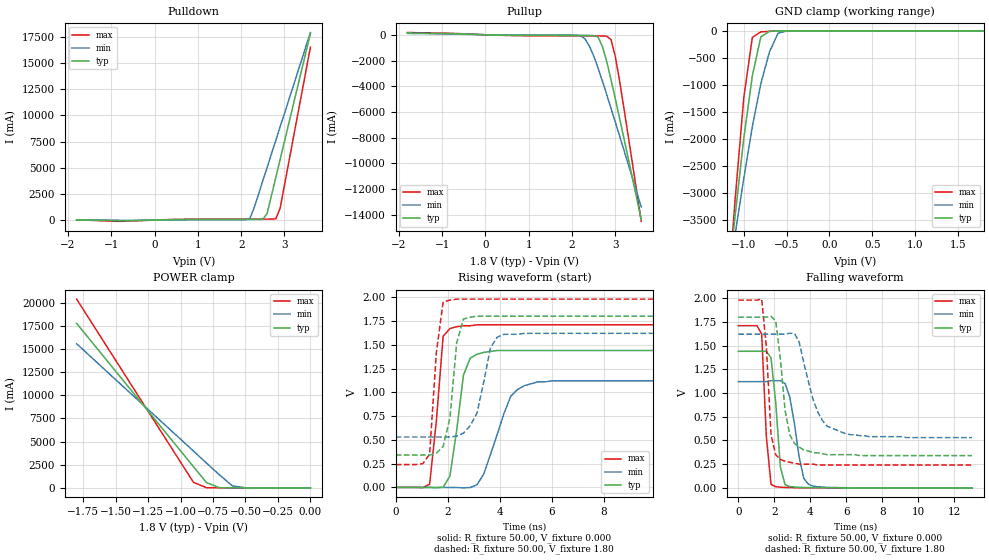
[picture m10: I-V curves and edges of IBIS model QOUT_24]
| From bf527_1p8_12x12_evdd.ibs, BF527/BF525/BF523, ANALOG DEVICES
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|   Model prw1624cdg_25
[Model]   QOUT_24
Model_type   I/O
Polarity   Non-Inverting
Enable   Active-Low
Vinl =   0.70V
Vinh =   1.00V
Vmeas =   1.20V
Cref =  50.00pF
Rref =   1.00M
Vref =  0.000V
C_comp   4.39pF   3.96pF   4.83pF
[Temperature Range]   25.00   0.12k   -40.00
[Voltage Range]   1.80V   1.62V   1.98V
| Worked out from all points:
|   slope of the pulldown table from 0 to 0.27 V, typ, clamps not added: 11.3 ohm
|   slope of the pullup table from 0 to 0.27 V, typ, clamps not added: 11.8 ohm
|   GND clamp passes 1 mA (typ) near -0.53 V on its own axis
|   POWER clamp passes 1 mA (typ) near -0.53 V on its own axis
|   rising waveform, R_fixture 50.00, V_fixture 0.000: 20-80 % time 416ps typ, 844ps min, 335ps max; typ from 0 V to 1.44 V
|   rising waveform, R_fixture 50.00, V_fixture 1.80: 20-80 % time 341ps typ, 535ps min, 306ps max; typ from 0.34 V to 1.8 V
|   falling waveform, R_fixture 50.00, V_fixture 0.000: 20-80 % time 373ps typ, 580ps min, 302ps max; typ from 1.44 V to 0 V
|   falling waveform, R_fixture 50.00, V_fixture 1.80: 20-80 % time 544ps typ, 1.03ns min, 326ps max; typ from 1.8 V to 0.34 V
[Pulldown]
| voltage   I(typ)   I(min)   I(max)
-1.8V     -10mA      0A         -10mA
-800mV    -73.8mA    -22.2mA    -120mA
600mV     42.5mA     23.13mA    69.61mA
2.1V      51.24mA    33.46mA    88.37mA
2.2V      51.32mA    140mA      88.44mA
2.3V      51.78mA    1.16A      88.5mA
2.5V      68.44mA    3.74A      89.43mA
2.6V      620mA      5.02A      92.15mA
2.8V      4.05A      7.6A       110mA
2.9V      5.77A      8.89A      1.11A
3.6V      17.82A     17.91A     16.51A
[Pullup]
| voltage   I(typ)   I(min)   I(max)
-1.8V     140mA      110mA      170mA
2.2V      -52.05mA   -57.07mA   -84.56mA
2.3V      -52.58mA   -320mA     -84.78mA
2.4V      -54.8mA    -870mA     -85.04mA
2.5V      -62.21mA   -1.62A     -86.03mA
2.6V      -160mA     -2.56A     -89.83mA
2.7V      -880mA     -3.57A     -96.83mA
2.8V      -2.04A     -4.62A     -110mA
2.9V      -3.46A     -5.69A     -360mA
3V        -4.95A     -6.77A     -1.66A
3.1V      -6.49A     -7.86A     -3.59A
3.6V      -14.34A    -13.37A    -14.49A
[GND_clamp]
| voltage   I(typ)   I(min)   I(max)
-1.8V     -14.28A    -11.35A    -18.41A
-1.2V     -4.9A      -4.81A     -5.19A
-1.1V     -3.4A      -3.75A     -3.1A
-1V       -1.99A     -2.73A     -1.24A
-900mV    -830mA     -1.77A     -120mA
-800mV    -110mA     -970mA     -19.15mA
-700mV    -9.85mA    -390mA     -9.73mA
-600mV    -2.55mA    -42.82mA   -3.48mA
-500mV    -450uA     -4.35mA    -550uA
1.8V      150pA      1.58uA     73.18pA
[POWER_clamp]
| voltage   I(typ)   I(min)   I(max)
-1.8V     17.76A     15.56A     20.38A
-900mV    2.28A      3.97A      590mA
-800mV    570mA      2.68A      16.99mA
-700mV    17.03mA    1.4A       7.08mA
-600mV    2.36mA     210mA      2.77mA
-500mV    460uA      11.86mA    530uA
0V        150pA      7.78nA     85.42pA
[Ramp]
| variable   typ   min   max
dV/dt_r   0.86/0.39n   0.67/0.76n   1.02/0.25n
dV/dt_f   0.87/0.47n   0.65/0.92n   1.04/0.28n
R_load = 50.00
[Rising Waveform]
R_fixture = 50.00
V_fixture = 0.000
V_fixture_min = 0.000
V_fixture_max = 0.000
L_fixture = 0.000H
C_fixture = 0.000F
| time   V(typ)   V(min)   V(max)
0s        0V         0V         0V
1.3ns     -450uV     54.95uV    33.4mV
1.56ns    -3.61mV    44.05uV    700mV
1.82ns    1.42mV     -63.47uV   1.59V
2.08ns    120mV      -450uV     1.67V
2.6ns     1.18V      -4.67mV    1.7V
3.12ns    1.4V       27.95mV    1.71V
4.42ns    1.44V      960mV      1.71V
4.94ns    1.44V      1.07V      1.71V
13ns      1.44V      1.12V      1.71V
[Rising Waveform]
R_fixture = 50.00
V_fixture = 1.80
V_fixture_min = 1.62
V_fixture_max = 1.98
L_fixture = 0.000H
C_fixture = 0.000F
| time   V(typ)   V(min)   V(max)
0s        340mV      530mV      240mV
1.3ns     340mV      530mV      350mV
1.56ns    360mV      530mV      1.42V
1.82ns    430mV      530mV      1.95V
2.34ns    1.52V      540mV      1.98V
2.6ns     1.77V      570mV      1.98V
3.12ns    1.8V       780mV      1.98V
3.64ns    1.8V       1.47V      1.98V
4.16ns    1.8V       1.61V      1.98V
13ns      1.8V       1.62V      1.98V
[Falling Waveform]
R_fixture = 50.00
V_fixture = 0.000
V_fixture_min = 0.000
V_fixture_max = 0.000
L_fixture = 0.000H
C_fixture = 0.000F
| time   V(typ)   V(min)   V(max)
0s        1.44V      1.12V      1.71V
1.3ns     1.44V      1.12V      1.62V
1.56ns    1.44V      1.12V      540mV
1.82ns    1.37V      1.13V      36.31mV
2.34ns    220mV      1.13V      6.86mV
2.6ns     32.93mV    1.1V       4.63mV
2.86ns    13.22mV    960mV      2.85mV
3.64ns    3.95mV     100mV      980uV
3.9ns     3.23mV     38.19mV    650uV
13ns      3.92uV     -23.47uV   -6.64uV
[Falling Waveform]
R_fixture = 50.00
V_fixture = 1.80
V_fixture_min = 1.62
V_fixture_max = 1.98
L_fixture = 0.000H
C_fixture = 0.000F
| time   V(typ)   V(min)   V(max)
0s        1.8V       1.62V      1.98V
1.3ns     1.8V       1.62V      1.99V
1.56ns    1.8V       1.62V      1.49V
1.82ns    1.81V      1.62V      560mV
2.08ns    1.76V      1.62V      350mV
2.34ns    1.36V      1.62V      300mV
2.86ns    560mV      1.63V      270mV
3.64ns    400mV      1.32V      250mV
4.94ns    350mV      650mV      240mV
13ns      340mV      530mV      240mV
